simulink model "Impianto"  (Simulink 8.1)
settings: Solver=FixedStepDiscrete  StartTime=0.0  StopTime=10.0  FixedStep=Ts  RelTol=1e-3
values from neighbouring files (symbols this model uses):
  Ts = time(2)-time(1)    [TSC160720ProvaMatlab.m]
undefined symbols (not defined in the file or in its folder): A, polyval
libraries: simulink x1, cstblocks x1

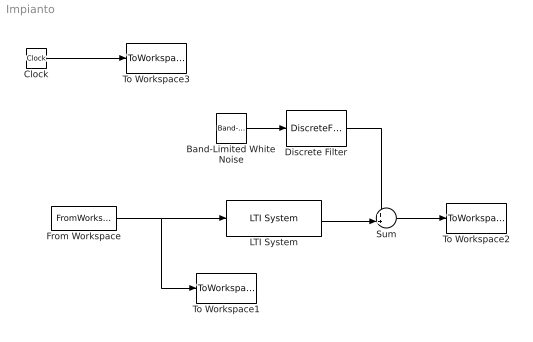
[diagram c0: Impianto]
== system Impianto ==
  Band-Limited White Noise : simulink/Sources/Band-Limited White Noise  Cov=noise_power  Ts=Ts  seed=[0]
  Clock : Clock
  Discrete Filter : DiscreteFilter  Numerator=[polyval(A,1)]  Denominator=A  SampleTime=Ts
  From Workspace : FromWorkspace  VariableName=[ti' ui']  SampleTime=0
  LTI System : cstblocks/LTI System  sys=Gd  IC=[]
  Sum : Sum  Inputs=++|
  To Workspace1 : ToWorkspace  VariableName=u  SampleTime=Ts
  To Workspace2 : ToWorkspace  VariableName=y  SampleTime=Ts
  To Workspace3 : ToWorkspace  VariableName=time  SampleTime=-1
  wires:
  From Workspace/1 -> To Workspace1/1, LTI System/1
  Sum/1 -> To Workspace2/1
  Clock/1 -> To Workspace3/1
  Band-Limited White Noise/1 -> Discrete Filter/1
  LTI System/1 -> Sum/2
  Discrete Filter/1 -> Sum/1
